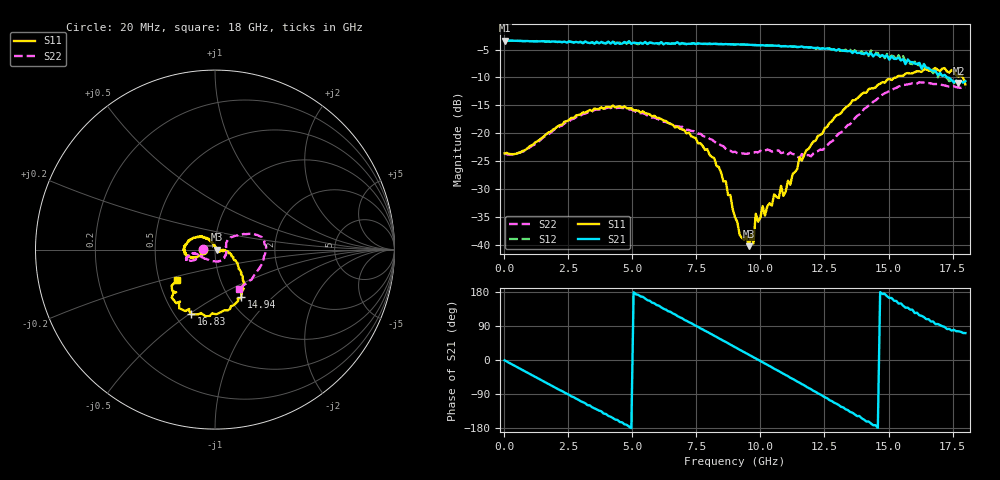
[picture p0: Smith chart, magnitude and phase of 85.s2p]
!Agilent Technologies,N5230A,US43500223,A.07.50.48
!Agilent N5230A: A.07.50.48
!Date: Sunday, January 10, 2016 20:13:25
!Correction: S11(Full 2 Port(1,2))
!S21(Full 2 Port(1,2))
!S12(Full 2 Port(1,2))
!S22(Full 2 Port(1,2))
!S2P File: Measurements: S11, S21, S12, S22:
# Hz S  dB  R 50
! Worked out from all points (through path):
!   201 points, 20 MHz to 18 GHz, reference 50 ohm
!   highest |S21| = -3.38 dB at 20 MHz (marker M1); lowest = -11.0 dB at 17.73 GHz (marker M2)
!   group delay of S21, straight-line fit = 103 ps
!   lowest |S11| = -40.3 dB at 9.549 GHz (marker M3), VSWR 1.02, Z = 51 - j0.123 ohm
!   |S11| at or under -10 dB: start of sweep to 15.3 GHz; 17.9 GHz to end of sweep
!   |S22| runs from -24.5 to -10.9 dB; largest |S21 - S12| = 0.049
!   S11 on the Smith chart (normalised r, x): 20 MHz: 0.88, +0.00; 14.94 GHz: 1.14, -0.66; 16.83 GHz: 0.60, -0.51; 18 GHz: 0.62, -0.23
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2e7  -23.65 179.6  -3.38 -0.8  -3.38 -0.7  -23.63 179.3
1.5483e9  -20.61 -157.4  -3.51 -56.8  -3.53 -57.0  -20.69 -153.9
3.0766e9  -16.26 -164.6  -3.88 -111.5  -3.80 -111.5  -16.59 -154.9
4.8746e9  -15.57 170.8  -3.51 -175.6  -3.60 -175.1  -15.72 -164.2
6.0433e9  -17.29 150.7  -3.92 143.2  -4.05 143.2  -17.54 -168.8
6.9423e9  -19.33 135.6  -3.87 110.4  -3.83 110.5  -18.84 -167.5
8.2009e9  -24.49 119.7  -3.97 64.2  -3.98 64.0  -21.49 -150.4
9.01e9  -35.08 84.7  -4.12 34.1  -4.07 34.1  -23.32 -118.4
9.5494e9  -40.28 -7.1  -4.13 14.1  -4.18 14.2  -23.63 -91.4
9.7292e9  -39.77 -20.6  -4.18 7.4  -4.21 7.4  -23.51 -82.8
9.8191e9  -34.46 -25.2  -4.20 4.1  -4.20 4.1  -23.39 -80.3
1.01787e10  -34.79 -25.4  -4.29 -9.1  -4.27 -9.4  -23.16 -64.3
1.0808e10  -29.46 -9.1  -4.45 -32.9  -4.41 -33.1  -23.58 -37.2
1.08979e10  -31.23 -0.4  -4.40 -36.2  -4.40 -36.4  -23.48 -31.6
1.20666e10  -21.52 -11.8  -4.72 -81.2  -4.68 -80.9  -23.67 18.3
1.36848e10  -14.08 -43.0  -5.28 -143.7  -5.13 -141.9  -17.33 34.6
1.49434e10  -10.42 -60.7  -6.05 168.1  -5.78 168.9  -12.69 22.2
1.50333e10  -10.26 -62.2  -6.83 163.6  -6.54 163.6  -12.42 20.6
1.60222e10  -9.10 -84.6  -7.54 124.0  -7.18 122.0  -11.16 7.6
1.68313e10  -8.30 -110.3  -8.88 94.6  -8.79 95.0  -11.19 -11.1
1.77303e10  -9.86 -132.3  -11.02 75.7  -11.08 73.7  -11.82 -46.6
1.8e10  -11.25 -141.1  -10.67 71.0  -10.94 71.1  -11.80 -58.4
